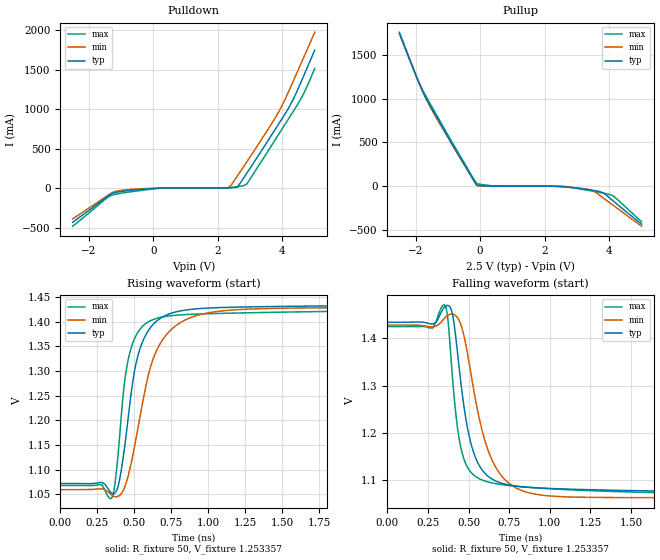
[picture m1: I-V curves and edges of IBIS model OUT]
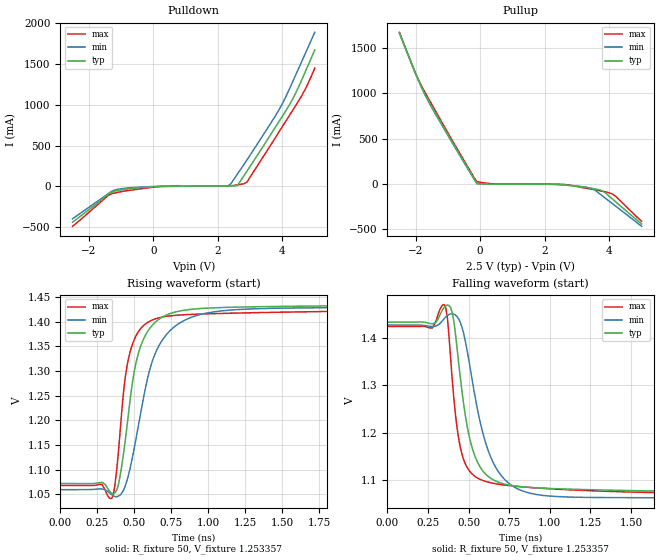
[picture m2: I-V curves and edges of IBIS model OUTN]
|   IBIS File of SG2520VHN D
|   LVDS, Vcc=2.5V, Io=3.5mA, fo>212.5MHz
[IBIS Ver]   3.2
[File Name]   sg2520vhn_hf_35m_25v.ibs
[File Rev]   1.0
[Date]   July 28, 2020
[Source]
Fairchild Ensigna Lab's Method
[Notes]
Created by Minoru Kozaki
[Disclaimer]
Seiko Epson Corporation makes no warranty with respect to the
information contained herein.
[Copyright]
Copyright(C) 2020, Seiko Epson Corporation. All rights reserved.
|   Component
[Component]   SG2520VHN
[Manufacturer]  Seiko Epson Corporation
[Package]
R_pkg   17.7m   NA   NA
L_pkg   235p   NA   NA
C_pkg   208f   NA   NA
[Pin]   signal_name   model_name   R_pin   L_pin   C_pin
1   OE/ST   NC
2   NC   NC
3   GND   GND
4   OUT   OUT   17.7m   235p   208f
5   OUTN   OUTN   10.4m   129p   221f
6   VCC   POWER
[Diff Pin] inv_pin  vdiff  tdelay_typ
4   5   0   0
| Models and submodels in the file (2): OUT (Output), OUTN (Output)
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|   Model OUT
[Model]   OUT
Model_type   Output
Polarity   Non-Inverting
Vref = 1.25
Vmeas = 1.25
Rref = 50
Cref = 0
C_comp   4.5p   4.5p   4.5p
[Temperature Range]   25   105   -40
[Voltage Range]   2.5   2.25   2.75
[Pullup Reference]   2.5   2.25   2.75
[Pulldown Reference]   0   0   0
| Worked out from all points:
|   slope of the pulldown table from 0 to 0.375 V, typ, clamps not added: 66.7 ohm
|   slope of the pullup table from 0 to 0.375 V, typ, clamps not added: 56.7 ohm
|   falling waveform, R_fixture 50, V_fixture 1.253357: 20-80 % time 111ps typ, 156ps min, 83.1ps max; typ from 1.43 V to 1.07 V
|   rising waveform, R_fixture 50, V_fixture 1.253357: 20-80 % time 126ps typ, 181ps min, 93.2ps max; typ from 1.07 V to 1.43 V
[Pullup]
-2.5V     1.749A     1.743A     1.76A
-2V       1.273A     1.279A     1.276A
-1.8V     1.098A     1.099A     1.112A
-1.6V     952.1mA    942.8mA    975.5mA
-800mV    438.8mA    429.4mA    456.9mA
-100mV    7.142mA    1.961mA    24.5mA
500mV     -3.427mA   -3.549mA   -2.439mA
2.6V      -11.44mA   -11.9mA    -5.6mA
3.4V      -45.12mA   -44.34mA   -54.74mA
3.8V      -79.15mA   -135.2mA   -81.16mA
4.1V      -166.6mA   -217.1mA   -111.5mA
5V        -438.9mA   -463.1mA   -410.7mA
[Pulldown]
-2.5V     -432.8mA   -390.3mA   -482.4mA
-1.4V     -96.72mA   -88.32mA   -111.1mA
-1.2V     -56.27mA   -43.75mA   -79.02mA
200mV     407uA      905.7uA    -657.1uA
2.3V      4.792mA    4.504mA    5.704mA
2.4V      5.746mA    32.97mA    8.506mA
2.6V      11.62mA    153.6mA    18.96mA
2.9V      193.4mA    336.4mA    56.07mA
3.9V      826.2mA    978.8mA    694.6mA
4.3V      1.1A       1.326A     952.1mA
4.6V      1.37A      1.604A     1.155A
5V        1.751A     1.976A     1.519A
[Falling Waveform]
R_fixture = 50
V_fixture = 1.253357
V_fixture_min = 1.243776
V_fixture_max = 1.246909
0s        1.434V     1.428V     1.425V
280ps     1.43V      1.425V     1.422V
350ps     1.466V     1.442V     1.472V
380ps     1.469V     1.451V     1.414V
420ps     1.407V     1.449V     1.245V
470ps     1.26V      1.408V     1.145V
590ps     1.118V     1.196V     1.099V
720ps     1.091V     1.101V     1.089V
1.1ns     1.08V      1.064V     1.079V
4ns       1.072V     1.06V      1.068V
[Rising Waveform]
R_fixture = 50
V_fixture = 1.253357
V_fixture_min = 1.243776
V_fixture_max = 1.246909
0s        1.072V     1.059V     1.068V
340ps     1.054V     1.05V      1.041V
380ps     1.058V     1.045V     1.101V
430ps     1.138V     1.061V     1.269V
470ps     1.236V     1.102V     1.339V
540ps     1.347V     1.211V     1.385V
650ps     1.401V     1.342V     1.406V
820ps     1.422V     1.399V     1.414V
1.15ns    1.429V     1.423V     1.417V
4ns       1.434V     1.428V     1.425V
[Ramp]
R_load = 50
dV/dt_r   0.21762/126.32p   0.22073/179.99p   0.21480/93.88p
dV/dt_f   0.21762/111.19p   0.22073/155.73p   0.21480/83.04p
|   Model OUTN
[Model]   OUTN
Model_type   Output
Polarity   Inverting
Vref = 1.25
Vmeas = 1.25
Rref = 50
Cref = 0
C_comp   4.5p   4.5p   4.5p
[Temperature Range]   25   105   -40
[Voltage Range]   2.5   2.25   2.75
[Pullup Reference]   2.5   2.25   2.75
[Pulldown Reference]   0   0   0
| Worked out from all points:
|   slope of the pulldown table from 0 to 0.375 V, typ, clamps not added: 66.6 ohm
|   slope of the pullup table from 0 to 0.375 V, typ, clamps not added: 56.8 ohm
|   falling waveform, R_fixture 50, V_fixture 1.253357: 20-80 % time 111ps typ, 155ps min, 82.9ps max; typ from 1.44 V to 1.07 V
|   rising waveform, R_fixture 50, V_fixture 1.253357: 20-80 % time 126ps typ, 181ps min, 93.3ps max; typ from 1.07 V to 1.43 V
[Pullup]
-2.5V     1.664A     1.661A     1.673A
-2V       1.214A     1.22A      1.219A
-1.7V     983.2mA    976.8mA    1.005A
-1V       545.8mA    535.9mA    564.2mA
-100mV    7.14mA     1.963mA    24.46mA
500mV     -3.427mA   -3.549mA   -2.441mA
2.6V      -11.45mA   -12.04mA   -5.602mA
3.4V      -45.67mA   -44.81mA   -55.11mA
3.6V      -58.19mA   -80.38mA   -67.76mA
3.8V      -79.71mA   -136.1mA   -81.94mA
4.1V      -167.8mA   -218.8mA   -112.1mA
5V        -442.7mA   -467.6mA   -413.2mA
[Pulldown]
-2.5V     -436.8mA   -394.1mA   -486.2mA
-1.4V     -97.55mA   -89.16mA   -111.7mA
-1.2V     -56.8mA    -44.15mA   -79.64mA
200mV     405.9uA    906.2uA    -660.6uA
2.3V      4.792mA    4.504mA    5.704mA
2.4V      5.744mA    31.85mA    8.499mA
2.6V      11.61mA    148.3mA    18.92mA
2.9V      186.7mA    324.7mA    54.34mA
4V        859.2mA    1.013A     732.7mA
4.4V      1.133A     1.352A     981.4mA
4.7V      1.395A     1.617A     1.183A
5V        1.666A     1.882A     1.444A
[Falling Waveform]
R_fixture = 50
V_fixture = 1.253357
V_fixture_min = 1.243776
V_fixture_max = 1.246909
0s        1.435V     1.428V     1.425V
280ps     1.431V     1.425V     1.423V
350ps     1.466V     1.442V     1.472V
390ps     1.465V     1.452V     1.356V
430ps     1.377V     1.446V     1.208V
480ps     1.237V     1.394V     1.134V
600ps     1.114V     1.184V     1.097V
720ps     1.091V     1.101V     1.089V
1.1ns     1.08V      1.063V     1.079V
4ns       1.072V     1.06V      1.068V
[Rising Waveform]
R_fixture = 50
V_fixture = 1.253357
V_fixture_min = 1.243776
V_fixture_max = 1.246909
0s        1.072V     1.059V     1.068V
350ps     1.052V     1.048V     1.043V
400ps     1.082V     1.048V     1.166V
430ps     1.141V     1.061V     1.268V
470ps     1.24V      1.102V     1.338V
540ps     1.348V     1.211V     1.385V
650ps     1.401V     1.342V     1.406V
820ps     1.422V     1.4V       1.413V
1.15ns    1.429V     1.423V     1.417V
4ns       1.434V     1.428V     1.425V
[Ramp]
R_load = 50
dV/dt_r   0.21740/126.19p  0.22051/179.24p  0.21457/93.91p
dV/dt_f   0.21740/110.47p  0.22051/154.30p  0.21457/82.55p
